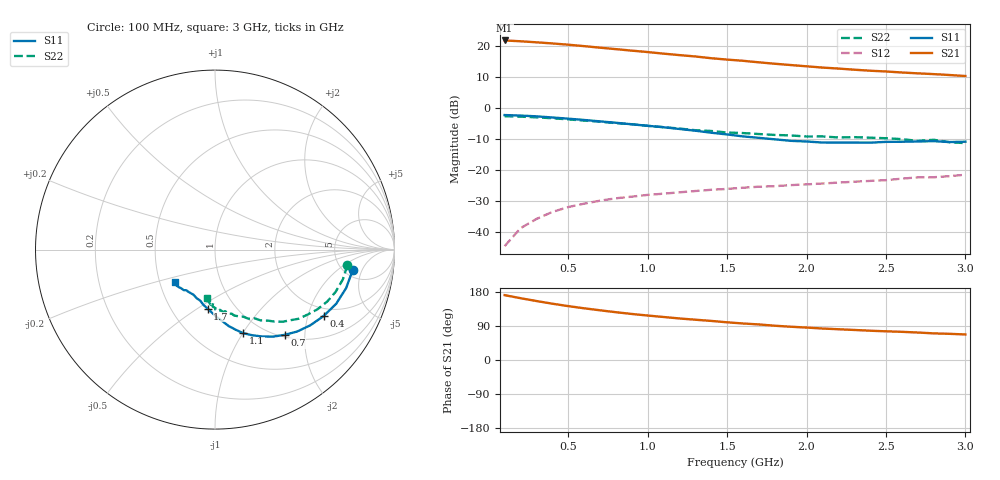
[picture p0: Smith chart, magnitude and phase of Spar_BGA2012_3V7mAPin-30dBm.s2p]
! Bias: Vs=Vc=3.00 V; Is=7.0 mA; Pin=-30 dBm
#  MHZ  S  MA  R 50
! Freq  S11  S21  S12  S22
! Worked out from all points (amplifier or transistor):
!   30 points, 100 MHz to 3 GHz, reference 50 ohm
!   highest |S21| = 22.0 dB at 100 MHz (marker M1)
!   |S21| within 3 dB of that: start of sweep to 838.8 MHz
!   unconditionally stable (mu >= 1): start of sweep to 137.7 MHz; 1.17 GHz to end of sweep
!   at 600 MHz: K = 0.66, MSG = 25.5 dB, |S12| = -30.9 dB
!   at 1.6 GHz: K = 1.27, MAG = 17.4 dB, |S12| = -25.7 dB
!   at 3 GHz: K = 1.58, MAG = 11.5 dB, |S12| = -21.5 dB
!   S11 on the Smith chart (normalised r, x): 100 MHz: 5.96, -3.39; 400 MHz: 1.69, -2.52; 700 MHz: 1.04, -1.58; 1.1 GHz: 0.82, -1.01; 1.7 GHz: 0.75, -0.55; 3 GHz: 0.60, -0.23
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100  0.776 -8.4  12.53 171.2  0.005839 84.9  0.7428 -6.7
200  0.7613 -16.4  12.15 163.1  0.0114 79.4  0.7315 -13.2
300  0.7395 -24.1  11.69 155.7  0.01609 76.4  0.712 -19.3
400  0.7091 -31.5  11.21 148.6  0.02091 72.2  0.6891 -24.9
500  0.6782 -38.5  10.69 142.2  0.02508 69.2  0.6599 -30.4
600  0.6463 -45.0  10.14 136.5  0.02848 66.0  0.6313 -34.9
700  0.6128 -50.8  9.568 131.2  0.03184 63.6  0.6054 -39.5
800  0.582 -56.5  9.061 126.1  0.03479 61.8  0.5737 -43.4
900  0.5495 -61.7  8.574 121.5  0.03699 60.5  0.5511 -46.8
1000  0.5199 -66.6  8.131 117.4  0.0395 58.9  0.5191 -50.5
1100  0.4923 -71.2  7.664 113.5  0.04134 58.7  0.4939 -53.2
1200  0.462 -75.4  7.254 109.6  0.04349 58.1  0.4696 -57.2
1300  0.4329 -79.8  6.897 106.3  0.04563 57.6  0.4409 -60.1
1500  0.3768 -88.4  6.137 99.5  0.04939 57.4  0.4047 -67.3
1600  0.35 -93.1  5.869 96.4  0.05162 57.3  0.3963 -70.0
1700  0.3318 -97.1  5.542 93.8  0.05362 57.5  0.3824 -73.8
1900  0.2966 -106.0  5.011 87.8  0.05687 57.3  0.3631 -78.8
2100  0.2783 -115.6  4.558 83.1  0.06042 57.7  0.3499 -82.6
2400  0.2769 -125.0  4.052 77.3  0.06658 58.1  0.3335 -89.8
2600  0.2867 -131.9  3.794 74.3  0.07251 61.0  0.3161 -92.6
2800  0.2933 -136.5  3.571 70.3  0.07629 60.2  0.3085 -94.4
3000  0.2873 -141.6  3.326 67.4  0.08386 61.4  0.2725 -99.5
